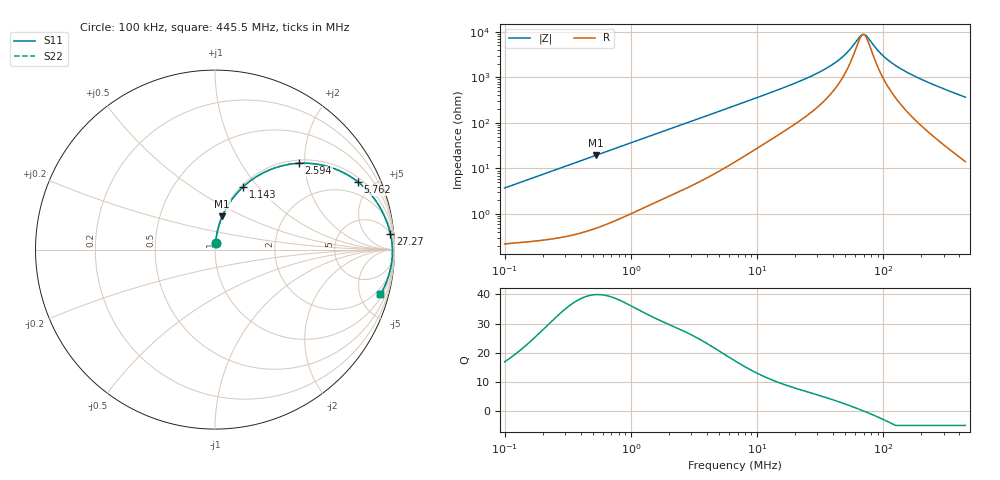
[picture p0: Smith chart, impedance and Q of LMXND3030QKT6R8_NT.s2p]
! LMXND3030QKT6R8_NT  S-PARAMETER MODEL  ( Standard Model )
! Model Generated by TAIYO YUDEN Corporation (https://www.yuden.co.jp/en/)
! Version 1.0
! TAIYO YUDEN Control No. 20250925
! Copyright(c) 2025 TAIYO YUDEN CO.,LTD. All Rights Reserved.
! Product Description (link to TY-COMPAS)
! https://ds.yuden.co.jp/TYCOMPAS/or/detail?pn=LMXND3030QKT6R8MNT&u=M
! Products Name : Inductors
! Characteristics :
!  Inductance : 6.8 [uH] , SRF(min) : 36 [MHz] , DC Resistance(max) : 0.192 [Ohm]
!  Rated Current : Saturation  870 [mA] , Temp Rise  1330 [mA] (40 [degC])
!  Case Size : 3.0 x 3.0 / 0.118 x 0.118 [mm/inch] , Thickness : 1.5 / 0.059 [mm/inch]
!  (Conditions: Temperature = 25 [degC] , DC Bias Current = 0 [A])
! External Node Assignments :
!  1  o---GGG---o  2
! GND o---------o GND
! Frequency Range : 0.1MHz  -  445.549718MHz  [ 402 STEP ]
# MHz S RI R 50
! Freq[MHz].  S11 Real  S11 Imag  S21 Real  S21 Imag  S12 Real  S12 Imag  S22 Real  S22 Imag
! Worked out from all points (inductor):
!   401 points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, 100 kHz to 445.5 MHz, reference 50 ohm
!   read as one part in series: L = 5.91 uH near 104.3 kHz
!   highest Q = 39.9 at 525.6 kHz (marker M1), where L = 5.85 uH
!   self-resonance near 68.71 MHz
!   S11 on the Smith chart (normalised r, x): 100 kHz: 1.00, +0.07; 1.143 MHz: 1.02, +0.83; 2.594 MHz: 1.07, +1.87; 5.762 MHz: 1.22, +4.13; 27.27 MHz: 5, +21; 445.5 MHz: 1.28, -7.31
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0.1  0.00358 0.037  0.9964 -0.037  0.9964 -0.037  0.00358 0.037
0.408498  0.0258 0.146  0.9742 -0.146  0.9742 -0.146  0.0258 0.146
0.525602  0.0403 0.1846  0.9597 -0.1846  0.9597 -0.1846  0.0403 0.1846
1.143352  0.1555 0.3483  0.8445 -0.3483  0.8445 -0.3483  0.1555 0.3483
1.668708  0.275 0.4308  0.725 -0.4308  0.725 -0.4308  0.275 0.4308
2.593864  0.4682 0.4811  0.5318 -0.4811  0.5318 -0.4811  0.4682 0.4811
3.707024  0.6345 0.4612  0.3655 -0.4612  0.3655 -0.4612  0.6345 0.4612
5.762254  0.7981 0.3759  0.2019 -0.3759  0.2019 -0.3759  0.7981 0.3759
6.81664  0.8426 0.3359  0.1574 -0.3359  0.1574 -0.3359  0.8426 0.3359
12.01907  0.9328 0.21  0.0672 -0.21  0.0672 -0.21  0.9328 0.21
27.26705  0.9773 0.0876  0.0227 -0.0876  0.0227 -0.0876  0.9773 0.0876
36.58892  0.9834 0.0567  0.0166 -0.0567  0.0166 -0.0567  0.9834 0.0567
45.14108  0.9861 0.037  0.0139 -0.037  0.0139 -0.037  0.9861 0.037
53.40106  0.9876 0.0222  0.0124 -0.0222  0.0124 -0.0222  0.9876 0.0222
64.51342  0.9885 0.00606  0.0115 -0.00606  0.0115 -0.00606  0.9885 0.00606
68.7095  0.9886 0.000732  0.0114 -0.000732  0.0114 -0.000732  0.9886 0.000732
74.73185  0.9888 -0.00639  0.0112 0.00639  0.0112 0.00639  0.9888 -0.00639
92.19941  0.9885 -0.0246  0.0115 0.0246  0.0115 0.0246  0.9885 -0.0246
111.3854  0.9875 -0.0418  0.0125 0.0418  0.0125 0.0418  0.9875 -0.0418
140.3372  0.9851 -0.0649  0.0149 0.0649  0.0149 0.0649  0.9851 -0.0649
188.3147  0.9795 -0.0991  0.0205 0.0991  0.0205 0.0991  0.9795 -0.0991
445.5497  0.9221 -0.2494  0.0779 0.2494  0.0779 0.2494  0.9221 -0.2494
